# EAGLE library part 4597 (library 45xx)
8-bit bus compatible COUNTER/LATCH
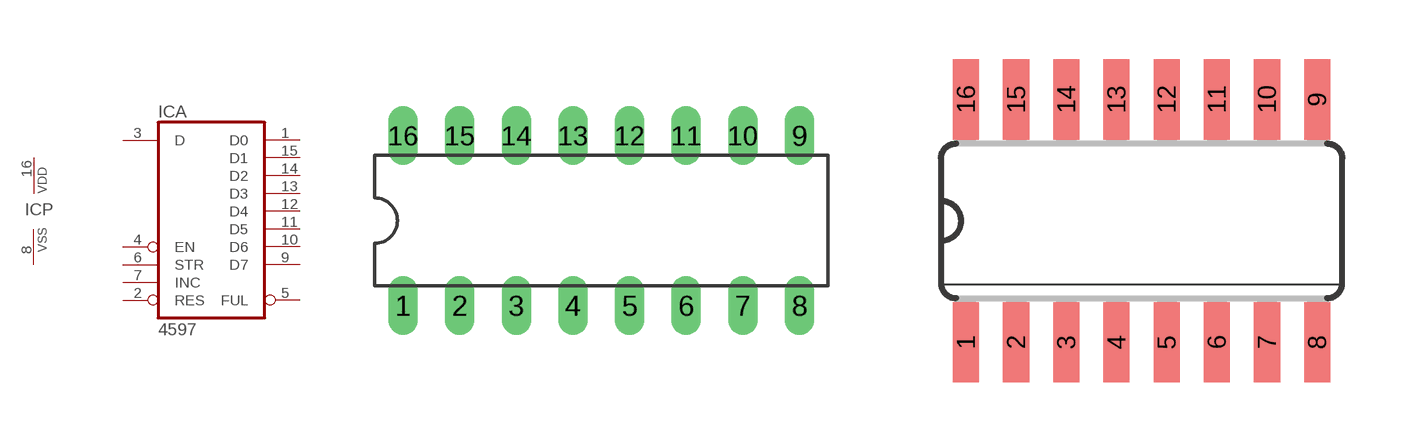
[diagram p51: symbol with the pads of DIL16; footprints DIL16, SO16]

Designator prefix IC; gates A=4597 P=PWRN

## 4597N  [DIL16]
1  A:D0  out
2  A:RES  in
3  A:D  in
4  A:EN  in
5  A:FUL  out
6  A:STR  in
7  A:INC  in
8  P:VSS  pwr
9  A:D7  out
10  A:D6  out
11  A:D5  out
12  A:D4  out
13  A:D3  out
14  A:D2  out
15  A:D1  out
16  P:VDD  pwr

## 4597D  [SO16]
Pads as for DIL16

## Footprint DIL16 (pad centres in mm)
Dual In Line Package
drill 0.813 long: 1 -8.89,-3.81; 2 -6.35,-3.81; 3 -3.81,-3.81; 4 -1.27,-3.81; 5 1.27,-3.81; 6 3.81,-3.81; 7 6.35,-3.81; 8 8.89,-3.81; 9 8.89,3.81; 10 6.35,3.81; 11 3.81,3.81; 12 1.27,3.81; 13 -1.27,3.81; 14 -3.81,3.81; 15 -6.35,3.81; 16 -8.89,3.81

## Footprint SO16 (pad centres in mm)
Small Outline package 150 mil
smd 0.66 x 2.032: 1 -4.445,-3.073; 2 -3.175,-3.073; 3 -1.905,-3.073; 4 -0.635,-3.073; 5 0.635,-3.073; 6 1.905,-3.073; 7 3.175,-3.073; 8 4.445,-3.073; 9 4.445,3.073; 10 3.175,3.073; 11 1.905,3.073; 12 0.635,3.073; 13 -0.635,3.073; 14 -1.905,3.073; 15 -3.175,3.073; 16 -4.445,3.073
